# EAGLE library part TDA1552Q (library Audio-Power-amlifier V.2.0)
The TDA1552Q is an integrated class-B output amplifier in a 13-lead single-in-line (SIL) plastic power package. The circuit contains 2 x 22 W amplifiers in Bridge Tied Load (BTL) configuration. The device is primarily developed for car radio applications.
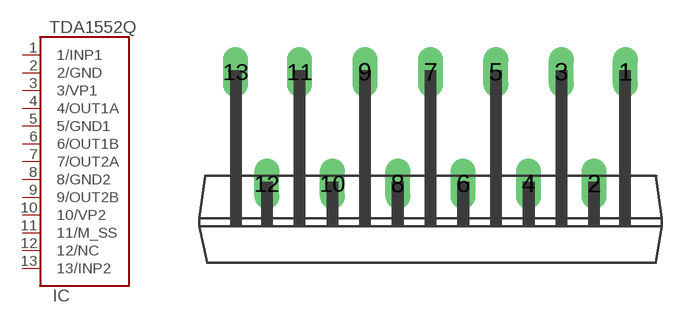
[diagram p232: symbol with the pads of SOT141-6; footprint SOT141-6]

Designator prefix IC

## TDA1552Q  [SOT141-6]
1  1/INP1
2  2/GND  pwr
3  3/VP1  pwr
4  4/OUT1A  out
5  5/GND1  pwr
6  6/OUT1B  out
7  7/OUT2A  out
8  8/GND2  pwr
9  9/OUT2B  out
10  10/VP2  pwr
11  11/M_SS  in
12  12/NC  nc
13  13/INP2  in

## Footprint SOT141-6 (pad centres in mm)
drill 0.8 long: 1 10.12,5.8; 2 8.5,0; 3 6.8,5.8; 4 5.1,0; 5 3.4,5.8; 6 1.7,0; 7 0,5.8; 8 -1.7,0; 9 -3.4,5.8; 10 -5.1,0; 11 -6.8,5.8; 12 -8.5,0; 13 -10.12,5.8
